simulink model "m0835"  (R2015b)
settings: Solver=ode3  StartTime=0.0  StopTime=10.0  RelTol=1e-3

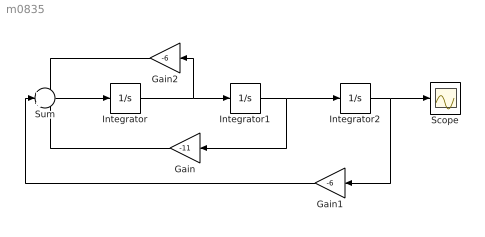
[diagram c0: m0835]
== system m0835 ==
  Gain : Gain  Gain=-11
  Gain1 : Gain  Gain=-6
  Gain2 : Gain  Gain=-6
  Integrator : Integrator  InitialCondition=1
  Integrator1 : Integrator
  Integrator2 : Integrator
  Scope : Scope
  Sum : Sum  Inputs=+++
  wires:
  Integrator2/1 -> Gain1/1, Scope/1
  Sum/1 -> Integrator/1
  Integrator/1 -> Gain2/1, Integrator1/1
  Integrator1/1 -> Gain/1, Integrator2/1
  Gain1/1 -> Sum/2
  Gain/1 -> Sum/3
  Gain2/1 -> Sum/1
